| IBIS file stm32wba52_a54_ufqfpn48.ibs
[IBIS ver] 4.2
[File name] stm32wba52_a54_ufqfpn48.ibs
[File Rev] 1.2
[Date] 22-05-2024
[Source] Data Created at STMicroelectronics
[Notes]  File originated from ELDO simulations.
[Disclaimer]  This information is for modeling purpose only and is
   not guaranteed. The information is subject to change without
   notice.
[Copyright] Copyright 2024 STMicroelectronics Inc.
|   Component stm32wba52_a54_ufqfpn48
[Component] stm32wba52_a54_ufqfpn48
[Manufacturer] STMicroelectronics
[Package]
| variable   typ   min   max
R_pkg  0  NA  NA
L_pkg  0  NA  NA
C_pkg  0  NA  NA
[Pin]   signal_name   model_name
0  VSS  gnd
1  PB12  io8_ft_100m_v33
2  PB11  io8_ft_100m_v33
3  PA8  io8_ft_100m_v33
4  PA7  io8_ft_100m_i2c_v33
5  PA6  io8_ft_100m_i2c_v33
6  VDDA  nc
7  PA5  io8_ft_100m_v33
8  PA3  io8_ft_100m_v33
9  PB10  io8_ft_100m_v33
10  PA2  io8_ft_100m_v33
11  VDD  power
12  PA1  io8_ft_100m_v33
13  PA0  io8_ft_100m_v33
14  PB9  io8_ft_100m_v33
15  PB8  io8_ft_100m_v33
16  PC15-OSC32_OUT  io8_ft_100m_tamp
17  PC14-OSC32_IN  io8_ft_100m_tamp
18  PC13  io8_ft_100m_v33
19  PB7  io8_ft_100m_v33
20  PB6  io8_ft_100m_v33
21  PB5  io8_ft_100m_v33
22  VDD  power
23  PB4  io8_ft_100m_v33
24  PB3  io8_ft_100m_i2c_v33
25  PA15  io8_ft_100m_i2c_v33
26  PA14  io8_ft_100m_v33
27  PA13  io8_ft_100m_v33
28  PA12  io8_ft_100m_v33
29  PA11  io8_ft_100m_v33
30  PB2  io8_ft_100m_i2c_v33
31  PB1  io8_ft_100m_i2c_v33
32  PB0  io8_ft_100m_v33
33  PB15  io8_ft_100m_v33
34  PH3-BOOT0  io8_ft_100m_v33
35  VDD  power
36  NRST  ioreset_v33
37  RF  nc
38  VDDHPA  nc
39  VDDRF  nc
40  OSC_OUT  nc
41  OSC_IN  nc
42  VDDRFPA  nc
43  VDD  power
44  VCAP  nc
45  PA10  io8_ft_100m_v33
46  PA9  io8_ft_100m_v33
47  PB14  io8_ft_100m_v33
48  PB13  io8_ft_100m_v33
[Package Model]   492-ufqfpn-7x7-48l-230116
[Pin Mapping]   pulldown_ref   pullup_ref   | Comment
0  gndio  nc
1  gndio  vddiom
2  gndio  vddiom
3  gndio  vddiom
4  gndio  vddiom
5  gndio  vddiom
6  nc  nc
7  gndio  vddiom
8  gndio  vddiom
9  gndio  vddiom
10  gndio  vddiom
11  nc  vddiom
12  gndio  vddiom
13  gndio  vddiom
14  gndio  vddiom
15  gndio  vddiom
16  gndio  vddiom
17  gndio  vddiom
18  gndio  vddiom
19  gndio  vddiom
20  gndio  vddiom
21  gndio  vddiom
22  nc  vddiom
23  gndio  vddiom
24  gndio  vddiom
25  gndio  vddiom
26  gndio  vddiom
27  gndio  vddiom
28  gndio  vddiom
29  gndio  vddiom
30  gndio  vddiom
31  gndio  vddiom
32  gndio  vddiom
33  gndio  vddiom
34  gndio  vddiom
35  nc  vddiom
36  gndio  vddiom
37  nc  nc
38  nc  nc
39  nc  nc
40  nc  nc
41  nc  nc
42  nc  nc
43  nc  vddiom
44  nc  nc
45  gndio  vddiom
46  gndio  vddiom
47  gndio  vddiom
48  gndio  vddiom
[Model Selector] io8_ft_100m_i2c_v33
io8_ft_100m_v33_ls_1v2  "GPIO_V33 100MHz - 5V tolerant - low speed - 1.2V range"
io8_ft_100m_v33_ls_1v8  "GPIO_V33 100MHz - 5V tolerant - low speed - 1.8V range"
io8_ft_100m_v33_ls_3v3  "GPIO_V33 100MHz - 5V tolerant - low speed - 3.3V range"
io8_ft_100m_v33_ms_1v2  "GPIO_V33 100MHz - 5V tolerant - med speed - 1.2V range"
io8_ft_100m_v33_ms_1v8  "GPIO_V33 100MHz - 5V tolerant - med speed - 1.8V range"
io8_ft_100m_v33_ms_3v3  "GPIO_V33 100MHz - 5V tolerant - med speed - 3.3V range"
io8_ft_100m_v33_fs_1v2  "GPIO_V33 100MHz - 5V tolerant - fast speed - 1.2V range"
io8_ft_100m_v33_fs_1v8  "GPIO_V33 100MHz - 5V tolerant - fast speed - 1.8V range"
io8_ft_100m_v33_fs_3v3  "GPIO_V33 100MHz - 5V tolerant - fast speed - 3.3V range"
io8_ft_100m_v33_hs_1v2  "GPIO_V33 100MHz - 5V tolerant - high speed - 1.2V range"
io8_ft_100m_v33_hs_1v8  "GPIO_V33 100MHz - 5V tolerant - high speed - 1.8V range"
io8_ft_100m_v33_hs_3v3  "GPIO_V33 100MHz - 5V tolerant - high speed - 3.3V range"
io8_ft_100m_i2c_v33_ls_1v2  "GPIO_V33 100MHz with I2C open-drain - 5V tolerant - low speed - 1.2V range"
io8_ft_100m_i2c_v33_ls_1v8  "GPIO_V33 100MHz with I2C open-drain - 5V tolerant - low speed - 1.8V range"
io8_ft_100m_i2c_v33_ls_3v3  "GPIO_V33 100MHz with I2C open-drain - 5V tolerant - low speed - 3.3V range"
io8_ft_100m_i2c_v33_ms_1v2  "GPIO_V33 100MHz with I2C open-drain - 5V tolerant - med speed - 1.2V range"
io8_ft_100m_i2c_v33_ms_1v8  "GPIO_V33 100MHz with I2C open-drain - 5V tolerant - med speed - 1.8V range"
io8_ft_100m_i2c_v33_ms_3v3  "GPIO_V33 100MHz with I2C open-drain - 5V tolerant - med speed - 3.3V range"
io8_ft_100m_i2c_v33_fs_1v2  "GPIO_V33 100MHz with I2C open-drain - 5V tolerant - fast speed - 1.2V range"
io8_ft_100m_i2c_v33_fs_1v8  "GPIO_V33 100MHz with I2C open-drain - 5V tolerant - fast speed - 1.8V range"
io8_ft_100m_i2c_v33_fs_3v3  "GPIO_V33 100MHz with I2C open-drain - 5V tolerant - fast speed - 3.3V range"
io8_ft_100m_i2c_v33_hs_1v2  "GPIO_V33 100MHz with I2C open-drain - 5V tolerant - high speed - 1.2V range"
io8_ft_100m_i2c_v33_hs_1v8  "GPIO_V33 100MHz with I2C open-drain - 5V tolerant - high speed - 1.8V range"
io8_ft_100m_i2c_v33_hs_3v3  "GPIO_V33 100MHz with I2C open-drain - 5V tolerant - high speed - 3.3V range"
io8_ft_100m_i2c_fmp_v33_3v3  "GPIO_V33 100MHz with I2C fm+ open-drain - 5V tolerant - low speed - 3.3V range"
[Model Selector] io8_ft_100m_tamp
io8_ft_100m_ls_1v2 "GPIO SPI - 5V tolerant - low speed - 1.2V range"
io8_ft_100m_ls_1v8 "GPIO SPI - 5V tolerant - low speed - 1.8V range"
io8_ft_100m_ls_3v3 "GPIO SPI - 5V tolerant - low speed - 3.3V range"
io8_ft_100m_ms_1v2 "GPIO SPI - 5V tolerant - med speed - 1.2V range"
io8_ft_100m_ms_1v8 "GPIO SPI - 5V tolerant - med speed - 1.8V range"
io8_ft_100m_ms_3v3 "GPIO SPI - 5V tolerant - med speed - 3.3V range"
io8_ft_100m_fs_1v2 "GPIO SPI - 5V tolerant - fast speed - 1.2V range"
io8_ft_100m_fs_1v8 "GPIO SPI - 5V tolerant - fast speed - 1.8V range"
io8_ft_100m_fs_3v3 "GPIO SPI - 5V tolerant - fast speed - 3.3V range"
io8_ft_100m_hs_1v2 "GPIO SPI - 5V tolerant - high speed - 1.2V range"
io8_ft_100m_hs_1v8 "GPIO SPI - 5V tolerant - high speed - 1.8V range"
io8_ft_100m_hs_3v3 "GPIO SPI - 5V tolerant - high speed - 3.3V range"
io8_ft_tamp_ls_1v2 "IO TAMPER_3V - 5V tolerant - low speed - 1.2V range"
io8_ft_tamp_ls_1v8 "IO TAMPER_3V - 5V tolerant - low speed - 1.8V range"
io8_ft_tamp_ls_3v3 "IO TAMPER_3V-  5V tolerant - low speed - 3.3V range"
io8_ft_tamp_ms_1v2 "IO TAMPER_3V - 5V tolerant - med speed - 1.2V range"
io8_ft_tamp_ms_1v8 "IO TAMPER_3V - 5V tolerant - med speed - 1.8V range"
io8_ft_tamp_ms_3v3 "IO TAMPER_3V - 5V tolerant - med speed - 3.3V range"
io8_ft_tamp_fs_1v2 "IO TAMPER_3V - 5V tolerant - fast speed - 1.2V range"
io8_ft_tamp_fs_1v8 "IO TAMPER_3V - 5V tolerant - fast speed - 1.8V range"
io8_ft_tamp_fs_3v3 "IO TAMPER_3V - 5V tolerant - fast speed - 3.3V range"
io8_ft_tamp_hs_1v2 "IO TAMPER_3V - 5V tolerant - high speed - 1.2V range"
io8_ft_tamp_hs_1v8 "IO TAMPER_3V - 5V tolerant - high speed - 1.8V range"
io8_ft_tamp_hs_3v3 "IO TAMPER_3V - 5V tolerant - high speed - 3.3V range"
[Model Selector] io8_ft_100m_v33
io8_ft_100m_v33_ls_1v2  "GPIO_V33 100MHz - 5V tolerant - low speed - 1.2V range"
io8_ft_100m_v33_ls_1v8  "GPIO_V33 100MHz - 5V tolerant - low speed - 1.8V range"
io8_ft_100m_v33_ls_3v3  "GPIO_V33 100MHz - 5V tolerant - low speed - 3.3V range"
io8_ft_100m_v33_ms_1v2  "GPIO_V33 100MHz - 5V tolerant - med speed - 1.2V range"
io8_ft_100m_v33_ms_1v8  "GPIO_V33 100MHz - 5V tolerant - med speed - 1.8V range"
io8_ft_100m_v33_ms_3v3  "GPIO_V33 100MHz - 5V tolerant - med speed - 3.3V range"
io8_ft_100m_v33_fs_1v2  "GPIO_V33 100MHz - 5V tolerant - fast speed - 1.2V range"
io8_ft_100m_v33_fs_1v8  "GPIO_V33 100MHz - 5V tolerant - fast speed - 1.8V range"
io8_ft_100m_v33_fs_3v3  "GPIO_V33 100MHz - 5V tolerant - fast speed - 3.3V range"
io8_ft_100m_v33_hs_1v2  "GPIO_V33 100MHz - 5V tolerant - high speed - 1.2V range"
io8_ft_100m_v33_hs_1v8  "GPIO_V33 100MHz - 5V tolerant - high speed - 1.8V range"
io8_ft_100m_v33_hs_3v3  "GPIO_V33 100MHz - 5V tolerant - high speed - 3.3V range"
[Model Selector] ioreset_v33
ioreset_v33_1v2 "Reset PAD. 5V tolerant. 1.2V range"
ioreset_v33_1v8 "Reset PAD. 5V tolerant. 1.8V range"
ioreset_v33_3v3 "Reset PAD. 5V tolerant. 3.3V range"
[Define Package Model]  492-ufqfpn-7x7-48l-230116
[Manufacturer]  Unknown
[OEM]  Unknown
[Description]  None
[Number Of Pins]  49
[Pin Numbers]
| Pin Num   Terminal Name
37 | RF
36 | NRST
13 | PA0
45 | PA10
29 | PA11
28 | PA12
27 | PA13
26 | PA14
25 | PA15
12 | PA1
10 | PA2
8 | PA3
7 | PA5
5 | PA6
4 | PA7
3 | PA8
46 | PA9
32 | PB0
9 | PB10
2 | PB11
1 | PB12
48 | PB13
47 | PB14
33 | PB15
31 | PB1
30 | PB2
24 | PB3
23 | PB4
21 | PB5
20 | PB6
19 | PB7
15 | PB8
14 | PB9
18 | PC13
17 | PC14-OSC32_IN
16 | PC15-OSC32_OUT
34 | PH3-BOOT0
44 | VCAP
43 | VDD
35 | VDD
11 | VDD
22 | VDD
6 | VDDA
38 | VDDHPA
39 | VDDRF
42 | VDDRFPA
0 | VSS
41 | OSC_IN
40 | OSC_OUT
[Model Data]
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[End Model Data]
[End Package Model]
|End [Component]
| Models and submodels in the file (52): io8_ft_100m_fs_1v2 (I/O), io8_ft_100m_fs_1v8 (I/O), io8_ft_100m_fs_3v3 (I/O), io8_ft_100m_hs_1v2 (I/O), io8_ft_100m_hs_1v8 (I/O), io8_ft_100m_hs_3v3 (I/O), io8_ft_100m_i2c_fmp_v33_3v3 (I/O_open_drain), io8_ft_100m_i2c_v33_fs_1v2 (I/O_open_drain), io8_ft_100m_i2c_v33_fs_1v8 (I/O_open_drain), io8_ft_100m_i2c_v33_fs_3v3 (I/O_open_drain), io8_ft_100m_i2c_v33_hs_1v2 (I/O_open_drain), io8_ft_100m_i2c_v33_hs_1v8 (I/O_open_drain), io8_ft_100m_i2c_v33_hs_3v3 (I/O_open_drain), io8_ft_100m_i2c_v33_ls_1v2 (I/O_open_drain), io8_ft_100m_i2c_v33_ls_1v8 (I/O_open_drain), io8_ft_100m_i2c_v33_ls_3v3 (I/O_open_drain), io8_ft_100m_i2c_v33_ms_1v2 (I/O_open_drain), io8_ft_100m_i2c_v33_ms_1v8 (I/O_open_drain), io8_ft_100m_i2c_v33_ms_3v3 (I/O_open_drain), io8_ft_100m_ls_1v2 (I/O), io8_ft_100m_ls_1v8 (I/O), io8_ft_100m_ls_3v3 (I/O), io8_ft_100m_ms_1v2 (I/O), io8_ft_100m_ms_1v8 (I/O), io8_ft_100m_ms_3v3 (I/O), io8_ft_100m_v33_fs_1v2 (I/O), io8_ft_100m_v33_fs_1v8 (I/O), io8_ft_100m_v33_fs_3v3 (I/O), io8_ft_100m_v33_hs_1v2 (I/O), io8_ft_100m_v33_hs_1v8 (I/O), io8_ft_100m_v33_hs_3v3 (I/O), io8_ft_100m_v33_ls_1v2 (I/O), io8_ft_100m_v33_ls_1v8 (I/O), io8_ft_100m_v33_ls_3v3 (I/O), io8_ft_100m_v33_ms_1v2 (I/O), io8_ft_100m_v33_ms_1v8 (I/O), io8_ft_100m_v33_ms_3v3 (I/O), io8_ft_tamp_fs_1v2 (I/O), io8_ft_tamp_fs_1v8 (I/O), io8_ft_tamp_fs_3v3 (I/O), io8_ft_tamp_hs_1v2 (I/O), io8_ft_tamp_hs_1v8 (I/O), io8_ft_tamp_hs_3v3 (I/O), io8_ft_tamp_ls_1v2 (I/O), io8_ft_tamp_ls_1v8 (I/O), io8_ft_tamp_ls_3v3 (I/O), io8_ft_tamp_ms_1v2 (I/O), io8_ft_tamp_ms_1v8 (I/O), io8_ft_tamp_ms_3v3 (I/O), ioreset_v33_1v2 (I/O_open_drain), ioreset_v33_1v8 (I/O_open_drain), ioreset_v33_3v3 (I/O_open_drain)
